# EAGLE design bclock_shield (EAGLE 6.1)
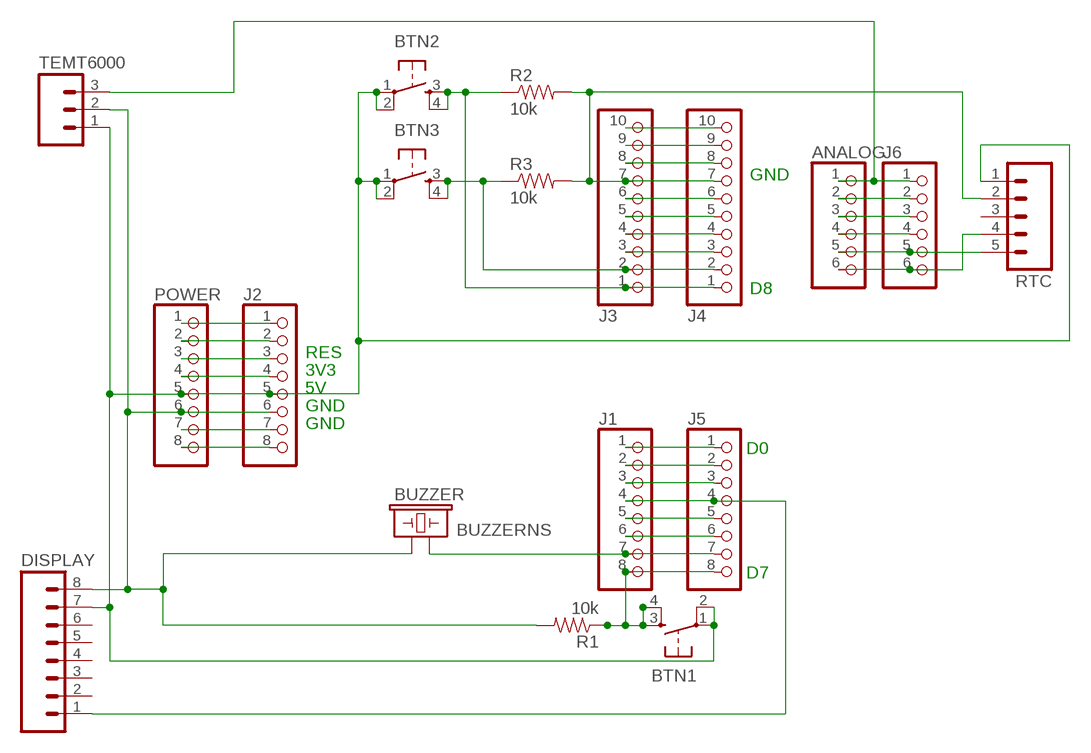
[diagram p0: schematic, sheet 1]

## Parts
ANALOG  PINHD-1X6  [1X06]
BTN1  TAC_SWITCHPTH  [TACTILE-PTH]
BTN2  TAC_SWITCHPTH  [TACTILE-PTH]
BTN3  TAC_SWITCHPTH  [TACTILE-PTH]
BUZZER  BUZZERNS  [BUZZER-12MM-NS]
DISPLAY  M081X08  [1X08]
J1  PINHD-1X8TH  [1X08-TH]
J2  PINHD-1X8TH  [1X08-TH]
J3  PINHD-1X10TH  [1X10-TH]
J4  PINHD-1X10TH  [1X10-TH]
J5  PINHD-1X8TH  [1X08-TH]
J6  PINHD-1X6  [1X06]
POWER  PINHD-1X8TH  [1X08-TH]
R1  10k  RESISTORPTH-1/4W  [AXIAL-0.4]
R2  10k  RESISTORPTH-1/4W  [AXIAL-0.4]
R3  10k  RESISTORPTH-1/4W  [AXIAL-0.4]
RTC  M05PTH  [1X05]
TEMT6000  M03PTH  [1X03]

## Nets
B+: BUZZER.- J1.7 J5.7
GND: BUZZER.+ DISPLAY.8 J2.6 POWER.6 R1.P$2 TEMT6000.2
N$1: J2.1 POWER.1
N$2: BTN2.3 BTN2.4 J3.1 J4.1 R2.P$1
N$3: J2.2 POWER.2
N$5: J3.4 J4.4
N$7: J3.3 J4.3
N$8: J1.1 J5.1
N$9: ANALOG.5 J6.5 RTC.5
N$10: J1.3 J5.3
N$11: DISPLAY.1 J1.4 J5.4
N$12: J1.5 J5.5
N$13: J1.6 J5.6
N$14: ANALOG.4 J6.4
N$15: BTN1.3 BTN1.4 J1.8 J5.8 R1.P$1
N$16: J2.4 POWER.4
N$18: J1.2 J5.2
N$19: ANALOG.2 J6.2
N$20: ANALOG.3 J6.3
N$21: J3.7 J4.7 R2.P$2 R3.P$2 RTC.2
N$22: BTN3.3 BTN3.4 J3.2 J4.2 R3.P$1
N$23: ANALOG.6 J6.6 RTC.4
N$26: J2.7 POWER.7
N$27: J2.8 POWER.8
N$28: J2.3 POWER.3
N$97: J3.6 J4.6
N$98: J3.5 J4.5
N$141: J3.9 J4.9
N$142: J3.10 J4.10
N$222: J3.8 J4.8
SIG: ANALOG.1 J6.1 TEMT6000.3
VCC: BTN1.1 BTN1.2 BTN2.1 BTN2.2 BTN3.1 BTN3.2 DISPLAY.7 J2.5 POWER.5 RTC.1 TEMT6000.1
Unconnected: DISPLAY.2 DISPLAY.3 DISPLAY.4 DISPLAY.5 DISPLAY.6 RTC.3

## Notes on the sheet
- GND
- D8
- RES
- 3V3
- 5V
- GND
- GND
- D0
- D7

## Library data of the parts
ANALOG J6 = pinhead:PINHD-1X6: PIN HEADER
BTN1-BTN3 = SparkFun:TAC_SWITCH: Momentary Switch Button commonly used for reset or general input. Spark Fun Electronics SKU : COM-00097
BUZZER = SparkFun:BUZZER: Buzzer 12mm
DISPLAY = SparkFun:M08: Header 8 Standard 8-pin 0.1" header. Use with straight break away headers (SKU : PRT-00116), right angle break away headers (PRT-00553), swiss pins (PRT-00743), machine pins (PRT-00117), and female headers (PRT-00115).
J1 J2 J5 POWER = SmartPrj:PINHD-1X8: PIN HEADER
J3 J4 = SmartPrj:PINHD-1X10: PIN HEADER
R1-R3 = SparkFun:RESISTOR: Resistor
RTC = SparkFun:M05: Header 5 Standard 5-pin 0.1" header. Use with straight break away headers (SKU : PRT-00116), right angle break away headers (PRT-00553), swiss pins (PRT-00743), machine pins (PRT-00117), and female headers (PRT-00115). Molex polarized connector foot print use with SKU : PRT-08230 with associated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
TEMT6000 = SparkFun:M03: Header 3 Standard 3-pin 0.1" header. Use with straight break away headers (SKU : PRT-00116), right angle break away headers (PRT-00553), swiss pins (PRT-00743), machine pins (PRT-00117), and female headers (PRT-00115). Molex polarized connector foot print use with SKU : PRT-08232 with associated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

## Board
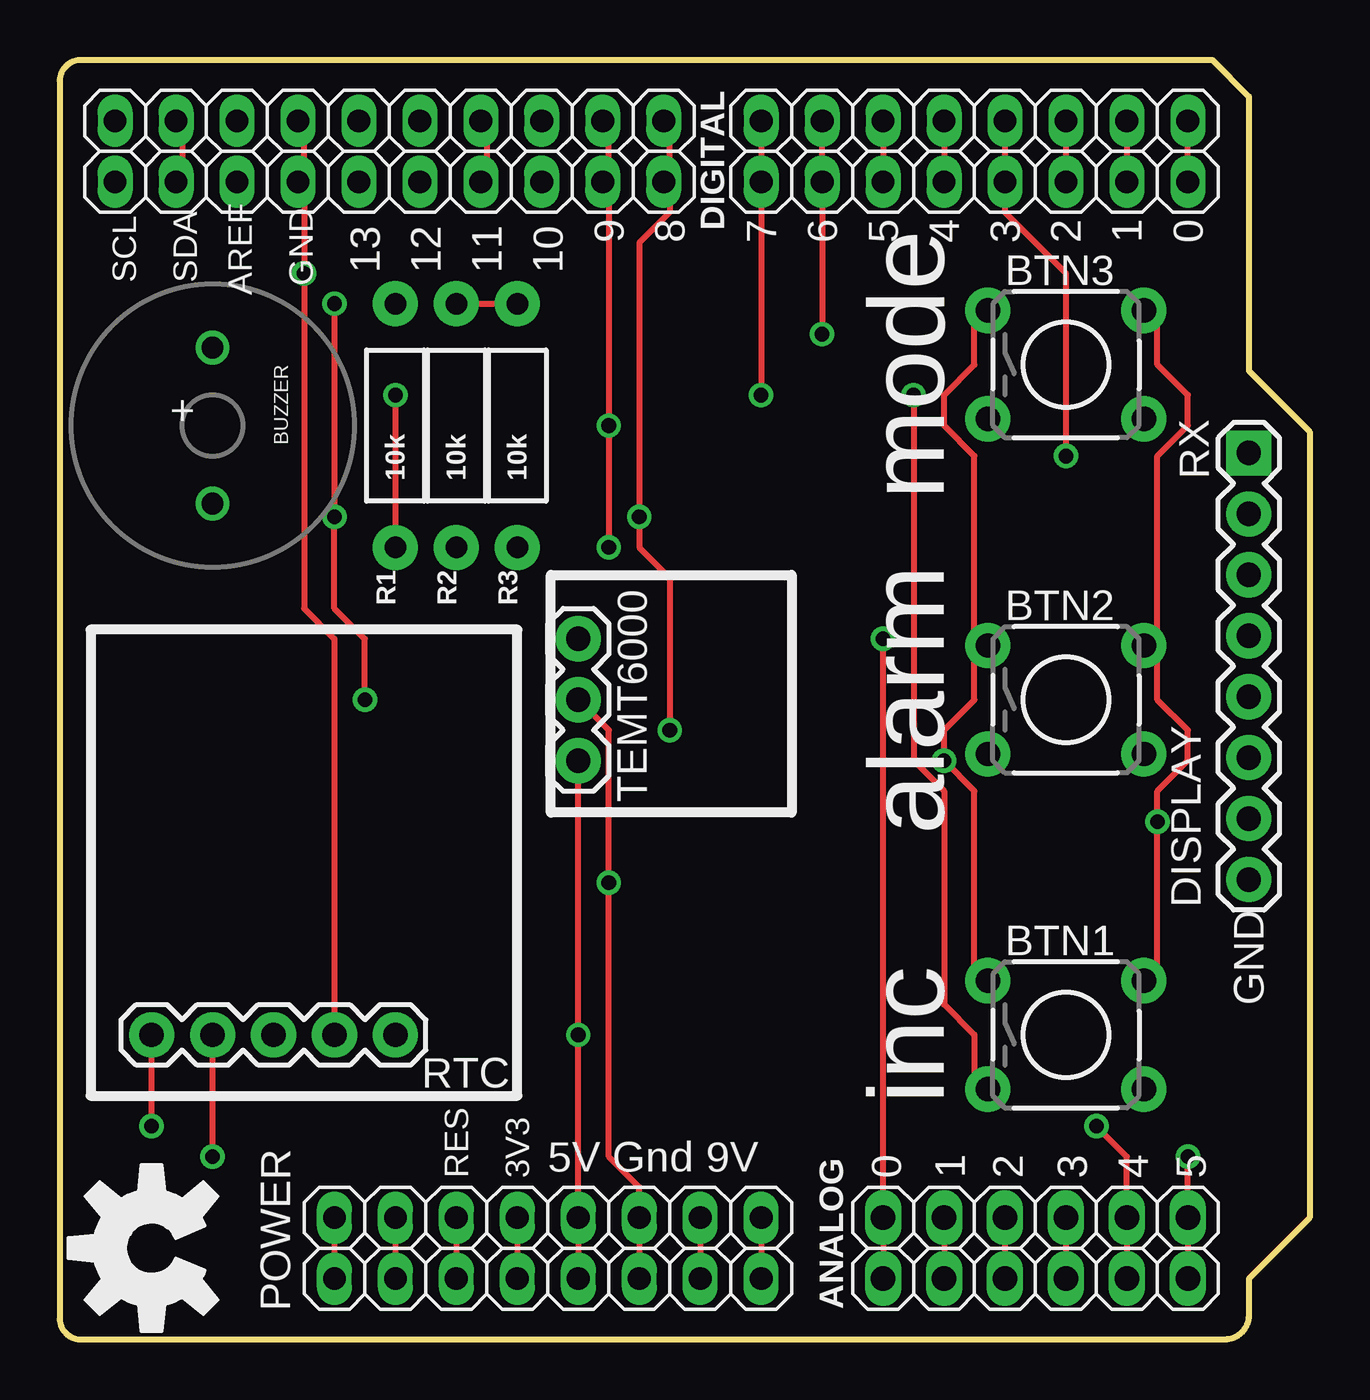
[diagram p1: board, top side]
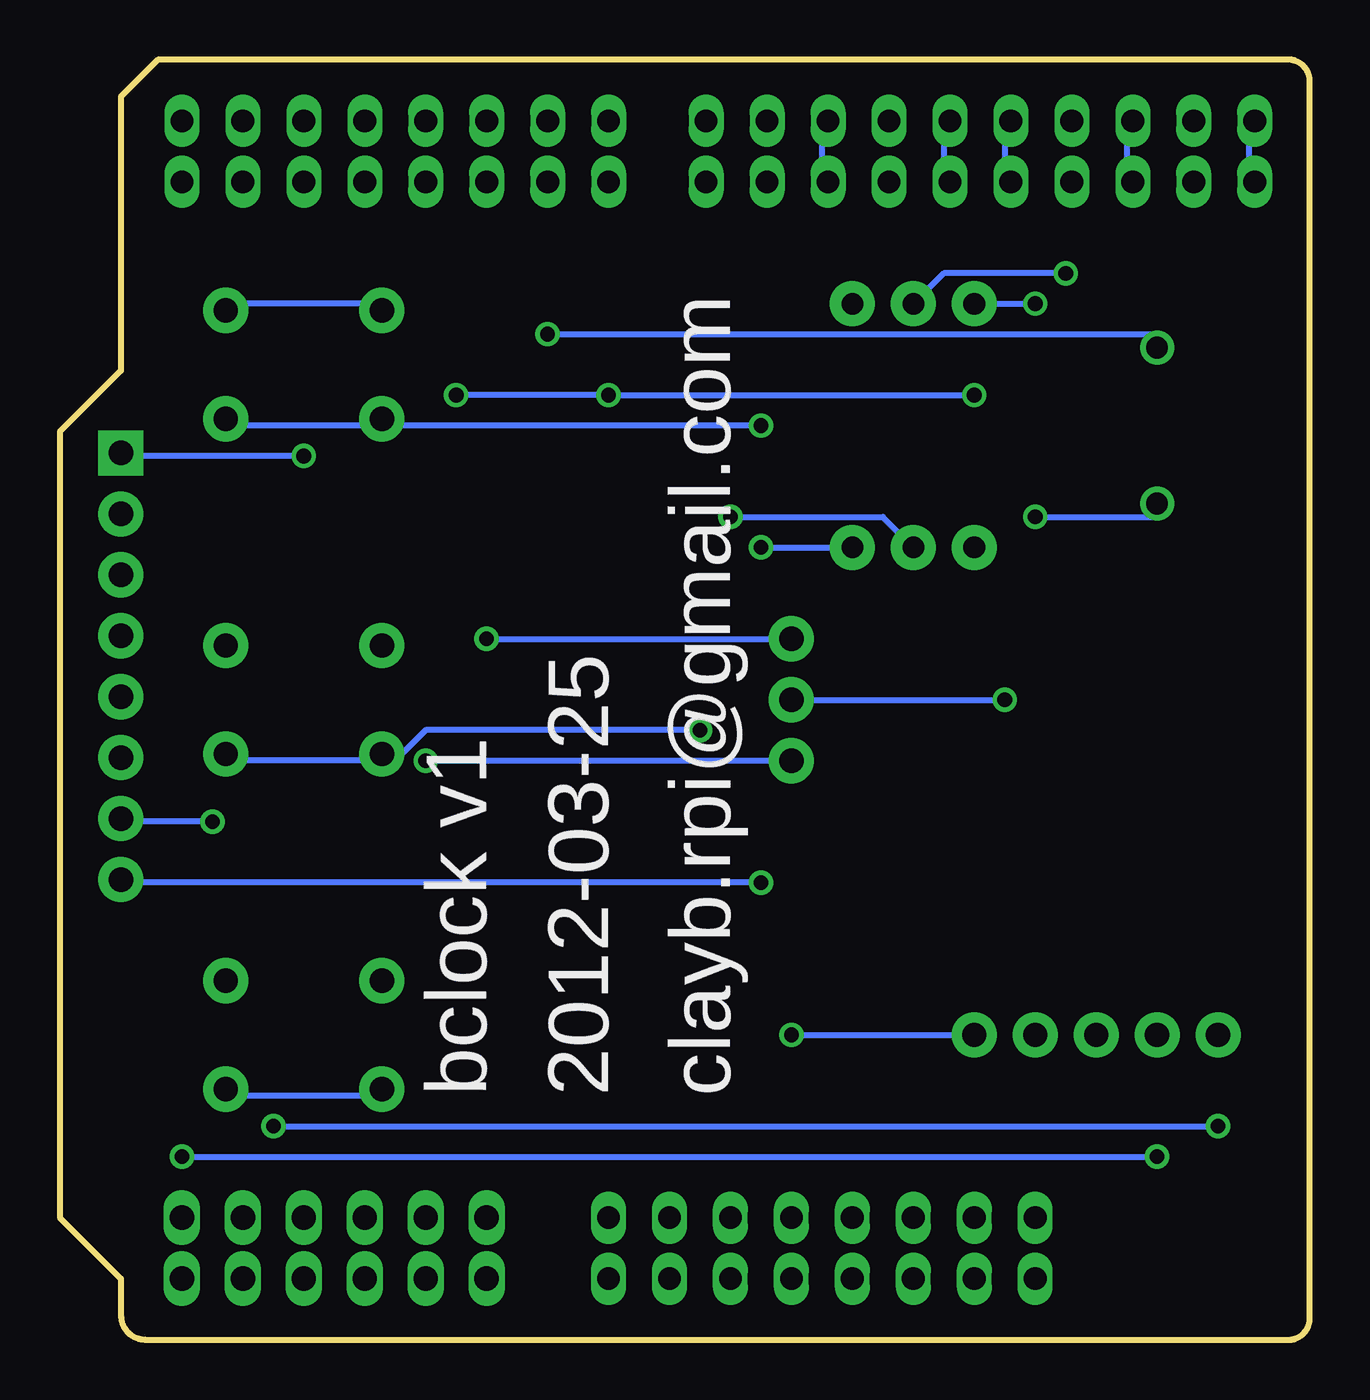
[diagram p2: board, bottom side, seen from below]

Size 52.08 x 53.34 mm. Coordinates in mm from the lower left corner, seen from the top.
Outline: 48.01,53.34 49.54,51.82 49.54,40.39 52.08,37.85 52.08,5.08 49.54,2.54 49.54,1 arc-90 48.54,0 0.75,0 arc-90 0.01,1 0.01,52.34 arc-90 0.75,53.34 48.01,53.34
Copper layers (1*16): Top 0.035mm / dielectric 1.5mm / Bottom 0.035mm
Design rules: minimum track width 10mil, minimum drill 24mil, track to track 8mil, track to pad 8mil, pad to pad 8mil, via to via 8mil, smd to smd 8mil, copper to edge 40mil, drill to drill 8mil, minimum pad ring 10mil, minimum via ring 8mil, stop-mask expansion 2mil, vias tented up to drill 0mil, thermal gap 10mil

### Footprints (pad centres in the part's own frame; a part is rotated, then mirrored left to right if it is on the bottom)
1X06 = drill 1.016 long: 1 -6.35,0; 2 -3.81,0; 3 -1.27,0; 4 1.27,0; 5 3.81,0; 6 6.35,0
TACTILE-PTH = drill 1.016 pad 1.88: 1 -3.251,2.261; 2 3.251,2.261; 3 -3.251,-2.261; 4 3.251,-2.261
BUZZER-12MM-NS = drill 0.9: + 3.25,0; - -3.25,0
1X08 = drill 1.016 pad 1.88 square: 1 0,0 | drill 1.016 pad 1.88: 2 2.54,0; 3 5.08,0; 4 7.62,0; 5 10.16,0; 6 12.7,0; 7 15.24,0; 8 17.78,0
1X08-TH = drill 0.95 pad 1.422 long: 1 -8.89,0; 2 -6.35,0; 3 -3.81,0; 4 -1.27,0; 5 1.27,0; 6 3.81,0; 7 6.35,0; 8 8.89,0
1X10-TH = drill 0.95 pad 1.422 long: 1 -11.43,0; 2 -8.89,0; 3 -6.35,0; 4 -3.81,0; 5 -1.27,0; 6 1.27,0; 7 3.81,0; 8 6.35,0; 9 8.89,0; 10 11.43,0
AXIAL-0.4 = drill 0.9 pad 1.88: P$1 -5.08,0; P$2 5.08,0
1X05 = drill 1.016 pad 1.88: 1 0,0; 2 2.54,0; 3 5.08,0; 4 7.62,0; 5 10.16,0
1X03 = drill 1.016 pad 1.88: 1 0,0; 2 2.54,0; 3 5.08,0

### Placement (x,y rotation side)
ANALOG  40.65,2.54 0 top
BTN1  41.92,12.7 0 top
BTN2  41.92,26.67 0 top
BTN3  41.92,40.64 0 top
BUZZER  6.36,38.1 270 top
DISPLAY  49.54,36.96 270 top
J1  38.11,50.8 180 top
J2  20.33,2.54 0 top
J3  13.72,50.8 180 top
J4  13.72,48.26 180 top
J5  38.11,48.26 180 top
J6  40.65,5.08 0 top
POWER  20.33,5.08 0 top
R1  13.98,38.1 90 top
R2  16.52,38.1 90 top
R3  19.06,38.1 90 top
RTC  13.98,12.7 180 top
TEMT6000  21.6,24.13 90 top
U$1  [OSHW-LOGO-L]  3.82,3.81 90 top

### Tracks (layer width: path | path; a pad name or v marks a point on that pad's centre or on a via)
B+  (via drill 0.61)
  Top 0.254: J1.7 J5.7 v31.76,41.91
  Bottom 0.254: v31.76,41.91 6.36,41.91 BUZZER.-
GND  (via drill 0.61)
  Top 0.254: J2.6 POWER.6 24.14,6.35 22.87,7.62 v22.87,19.05 22.87,25.4 TEMT6000.2 | v11.44,43.18 v11.44,34.29 11.44,30.48 12.71,29.21 v12.71,26.67
  Bottom 0.254: v11.44,34.29 6.36,34.29 BUZZER.+ | R1.P$2 v11.44,43.18 | v22.87,19.05 49.54,19.05 DISPLAY.8 | TEMT6000.2 v12.71,26.67
N$1
  Top 0.254: POWER.1 J2.1
N$2  (via drill 0.61)
  Top 0.254: 25.41,48.26 25.41,50.8 J3.1 | 25.41,48.26 25.41,46.99 24.14,45.72 v24.14,34.29 24.14,33.02 25.41,31.75 v25.41,25.4 | 25.41,48.26 J4.1
  Bottom 0.254: BTN2.4 44.46,24.13 39.38,24.13 BTN2.3 38.11,24.13 36.84,25.4 v25.41,25.4 | R2.P$1 17.79,34.29 v24.14,34.29
N$3
  Top 0.254: POWER.2 J2.2
N$5
  Top 0.254: J4.4 17.79,48.26 17.79,50.8 J3.4
N$7
  Bottom 0.254: J4.3 20.33,48.26 20.33,50.8 J3.3
N$8
  Top 0.254: J5.1 J1.1
N$9  (via drill 0.61)
  Top 0.254: ANALOG.5 J6.5 44.46,7.62 v43.19,8.89 | v3.82,8.89 RTC.5
  Bottom 0.254: v43.19,8.89 v3.82,8.89
N$10
  Top 0.254: J1.3 J5.3
N$11  (via drill 0.61)
  Top 0.254: J1.4 J5.4 39.38,46.99 41.92,44.45 v41.92,36.83
  Bottom 0.254: v41.92,36.83 49.54,36.83 DISPLAY.1
N$12
  Top 0.254: J1.5 J5.5
N$13
  Top 0.254: J1.6 J5.6
N$14
  Top 0.254: J6.4 ANALOG.4
N$15  (via drill 0.61)
  Top 0.254: J1.8 J5.8 v29.22,39.37 | v13.98,39.37 R1.P$1 | v35.57,39.37 35.57,24.13 36.84,22.86 36.84,13.97 38.11,12.7 38.11,10.16 BTN1.3
  Bottom 0.254: BTN1.4 44.46,10.16 39.38,10.16 BTN1.3 | v13.98,39.37 v29.22,39.37 v35.57,39.37
N$16
  Top 0.254: POWER.4 J2.4
N$18
  Top 0.254: J1.2 J5.2
N$19
  Top 0.254: J6.2 ANALOG.2
N$20
  Top 0.254: J6.3 ANALOG.3
N$21  (via drill 0.61)
  Top 0.254: R2.P$2 R3.P$2 | 10.17,48.26 10.17,50.8 J3.7 | RTC.2 11.44,29.21 10.17,30.48 v10.17,44.45 10.17,48.26 | 10.17,48.26 J4.7
  Bottom 0.254: R2.P$2 15.25,44.45 v10.17,44.45
N$22  (via drill 0.61)
  Top 0.254: 22.87,48.26 22.87,50.8 J3.2 | 22.87,48.26 v22.87,38.1 v22.87,33.02 | 22.87,48.26 J4.2
  Bottom 0.254: BTN3.4 44.46,38.1 39.38,38.1 BTN3.3 38.11,38.1 v22.87,38.1 | v22.87,33.02 R3.P$1
N$23  (via drill 0.61)
  Top 0.254: ANALOG.6 J6.6 v47,7.62 | v6.36,7.62 RTC.4
  Bottom 0.254: v47,7.62 v6.36,7.62
N$26
  Top 0.254: POWER.7 J2.7
N$27
  Top 0.254: POWER.8 J2.8
N$28
  Top 0.254: POWER.3 J2.3
N$97
  Bottom 0.254: J4.6 12.71,48.26 12.71,50.8 J3.6
N$98
  Bottom 0.254: J4.5 15.25,48.26 15.25,50.8 J3.5
N$141
  Top 0.254: J4.9 5.09,48.26 5.09,50.8 J3.9
  Bottom 0.254: 5.09,48.26 J4.9 | 5.09,50.8 J3.9
N$142
  Bottom 0.254: J4.10 2.55,48.26 2.55,50.8 J3.10
N$222
  Bottom 0.254: J4.8 7.63,48.26 7.63,50.8 J3.8
SIG  (via drill 0.61)
  Top 0.254: ANALOG.1 J6.1 v34.3,29.21
  Bottom 0.254: v34.3,29.21 TEMT6000.3
VCC  (via drill 0.61)
  Top 0.254: J2.5 POWER.5 v21.6,12.7 TEMT6000.1 | 45.73,29.21 45.73,26.67 47,25.4 47,24.13 45.73,22.86 v45.73,21.59 45.73,15.24 BTN1.2 | 45.73,29.21 45.73,36.83 47,38.1 47,39.37 45.73,40.64 45.73,43.18 BTN3.2 | 45.73,29.21 BTN2.2 | 38.11,29.21 38.11,26.67 36.84,25.4 v36.84,24.13 38.11,22.86 38.11,15.24 BTN1.1 | 38.11,29.21 38.11,36.83 36.84,38.1 36.84,39.37 38.11,40.64 38.11,43.18 BTN3.1 | 38.11,29.21 BTN2.1
  Bottom 0.254: v45.73,21.59 49.54,21.59 DISPLAY.7 | v21.6,12.7 RTC.1 | v36.84,24.13 TEMT6000.1 | BTN3.2 44.46,43.18 39.38,43.18 BTN3.1

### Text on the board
tPlace: 9 | 8 | 7 | 6 | 5 | 4 | 3 | 2 | 1 | 0 | 13 | 12 | 11 | 10
tNames: DIGITAL | AREF | SCL | SDA | GND | mode | + | RX | alarm | GND | inc | RES | 3V3 | 5V Gnd 9V | 0 | 1 | 2 | 3 | 4 | 5
bNames: clayb.rpi@gmail.com | 2012-03-25 | bclock v1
